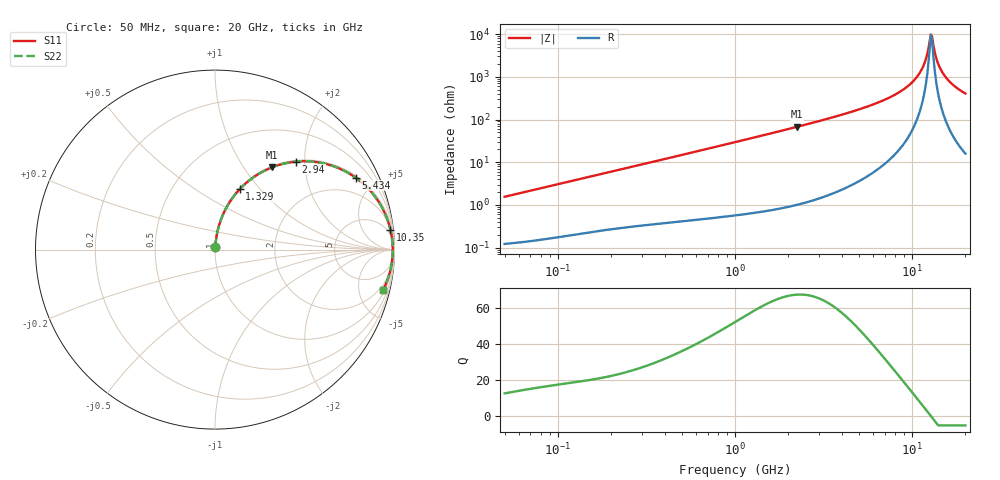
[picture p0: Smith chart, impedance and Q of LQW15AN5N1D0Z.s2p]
!Murata Part Number: LQW15AN5N1D0Z
!These Parameters are Measured in Series Mode Connection
!  o--[Z]--o
!Port1  Port2
!  o-------o
!Freq. Start=50[MHz] Stop=20[GHz], 401[Steps]
# Hz S RI R 50
!Freq.(Hz) S11(Real) S11(Imag) S21(Real) S21(Imag) S12(Real) S12(Imag) S22(Real) S22(Imag)
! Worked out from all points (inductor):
!   401 points, 50 MHz to 20 GHz, reference 50 ohm
!   read as one part in series: L = 4.91 nH near 51.52 MHz
!   highest Q = 67.2 at 2.245 GHz (marker M1), where L = 4.79 nH
!   self-resonance near 12.76 GHz
!   S11 on the Smith chart (normalised r, x): 50 MHz: 1.00, +0.03; 1.329 GHz: 1.01, +0.79; 2.94 GHz: 1.03, +1.81; 5.434 GHz: 1.09, +3.86; 10.35 GHz: 2, +17; 20 GHz: 1.32, -8.13
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5e7  0.00146 0.0154  0.9985 -0.0154  0.9985 -0.0154  0.00146 0.0154
1.364002e8  0.00383 0.0411  0.9962 -0.0411  0.9962 -0.0411  0.00383 0.0411
3.721004e8  0.0155 0.1082  0.9845 -0.1082  0.9845 -0.1082  0.0155 0.1082
1e9  0.0843 0.2684  0.9157 -0.2684  0.9157 -0.2684  0.0843 0.2684
1.329223e9  0.138 0.3365  0.862 -0.3365  0.862 -0.3365  0.138 0.3365
2.245319e9  0.3163 0.4576  0.6837 -0.4576  0.6837 -0.4576  0.3163 0.4576
2.728004e9  0.4114 0.4846  0.5886 -0.4846  0.5886 -0.4846  0.4114 0.4846
2.940159e9  0.4512 0.49  0.5488 -0.49  0.5488 -0.49  0.4512 0.49
5.433528e9  0.7833 0.4009  0.2167 -0.4009  0.2167 -0.4009  0.7833 0.4009
7.442007e9  0.9066 0.2741  0.0934 -0.2741  0.0934 -0.2741  0.9066 0.2741
9.041845e9  0.9558 0.1804  0.0442 -0.1804  0.0442 -0.1804  0.9558 0.1804
1.034674e10  0.9772 0.1119  0.0228 -0.1119  0.0228 -0.1119  0.9772 0.1119
1.166392e10  0.9877 0.0496  0.0123 -0.0496  0.0123 -0.0496  0.9877 0.0496
1.201863e10  0.989 0.0339  0.011 -0.0339  0.011 -0.0339  0.989 0.0339
1.257102e10  0.9901 0.0104  0.00987 -0.0104  0.00987 -0.0104  0.9901 0.0104
1.276073e10  0.9902 0.00254  0.00975 -0.00254  0.00975 -0.00254  0.9902 0.00254
1.314879e10  0.9901 -0.0132  0.0099 0.0132  0.0099 0.0132  0.9901 -0.0132
1.375312e10  0.9889 -0.0367  0.0111 0.0367  0.0111 0.0367  0.9889 -0.0367
1.417136e10  0.9875 -0.0524  0.0125 0.0524  0.0125 0.0524  0.9875 -0.0524
1.504638e10  0.9832 -0.0837  0.0168 0.0837  0.0168 0.0837  0.9832 -0.0837
1.696185e10  0.9686 -0.1454  0.0314 0.1454  0.0314 0.1454  0.9686 -0.1454
2e10  0.9351 -0.2276  0.0649 0.2276  0.0649 0.2276  0.9351 -0.2276
